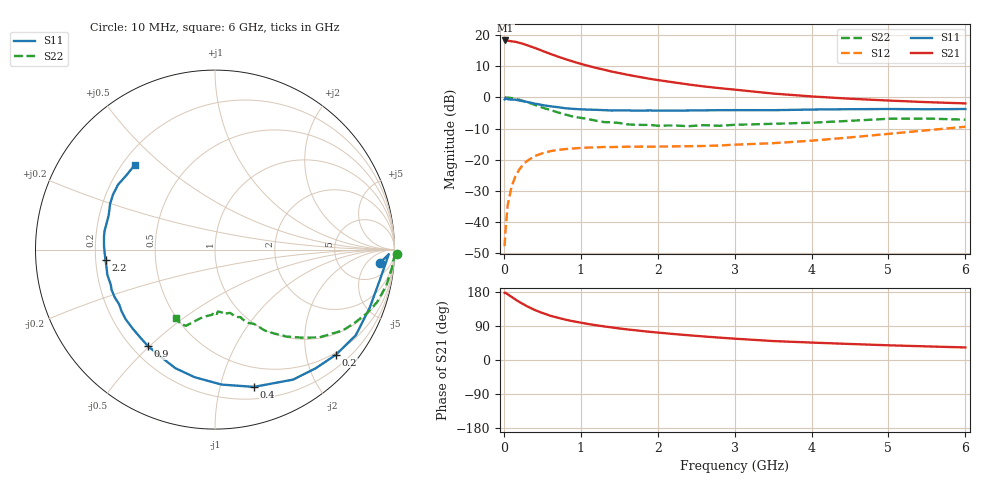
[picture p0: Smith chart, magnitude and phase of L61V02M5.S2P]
!  INFINEON TECHNOLOGIES Small Signal Semiconductors
! BFR380L3 , Si-NPN RF-Transistor in TSLP-3-1
!  Vce=1 V,  Ic=2.5 mA
! Common Emitter S-Parameters:  07. March 2005
#  GHz  S  MA  R  50
! f  S11  S21  S12  S22
! GHz  Mag  Ang  Mag  Ang  Mag  Ang  Mag  Ang
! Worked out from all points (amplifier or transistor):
!   36 points, 10 MHz to 6 GHz, reference 50 ohm
!   highest |S21| = 18.3 dB at 20 MHz (marker M1)
!   |S21| within 3 dB of that: start of sweep to 466.3 MHz
!   unconditionally stable (mu >= 1): 2.647 GHz to 4.82 GHz
!   at 250 MHz: K = 0.10, MSG = 19.4 dB, |S12| = -21.6 dB
!   at 1.4 GHz: K = 0.61, MSG = 12.1 dB, |S12| = -15.9 dB
!   at 6 GHz: K = 0.94, MSG = 3.7 dB, |S12| = -9.4 dB
!   S11 on the Smith chart (normalised r, x): 10 MHz: 13, -13; 200 MHz: 0.45, -2.61; 400 MHz: 0.31, -1.28; 900 MHz: 0.26, -0.49; 2.2 GHz: 0.24, -0.05; 6 GHz: 0.25, +0.41
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0.01  0.9239 -4.5  8.127 177.0  0.0041 84.9  1.013 -1.3
0.02  0.9687 -1.5  8.181 177.7  0.007 88.4  0.9989 -2.6
0.05  0.9335 -10.6  8.096 173.2  0.0187 84.8  0.9907 -6.1
0.1  0.9209 -20.6  7.929 166.6  0.0368 78.8  0.975 -11.9
0.15  0.918 -31.3  7.79 159.8  0.0539 73.1  0.9498 -17.9
0.2  0.8932 -40.9  7.512 153.3  0.0695 68.2  0.9178 -22.7
0.3  0.8451 -59.0  6.874 141.9  0.0951 58.7  0.8417 -32.4
0.4  0.7949 -74.2  6.225 132.2  0.1142 51.5  0.7594 -40.1
0.5  0.753 -87.2  5.583 124.2  0.1265 46.0  0.6878 -45.5
0.6  0.7199 -99.1  5.003 117.1  0.1369 41.2  0.6278 -50.5
0.7  0.6965 -108.5  4.518 111.6  0.1433 38.4  0.5755 -54.5
0.8  0.6693 -116.9  4.11 106.5  0.1481 35.7  0.531 -58.3
0.9  0.654 -125.0  3.748 102.2  0.1512 33.5  0.4904 -60.7
1.1  0.6355 -136.4  3.193 94.8  0.1565 31.0  0.4478 -65.6
1.3  0.6239 -146.6  2.784 88.7  0.16 29.8  0.4013 -69.4
1.6  0.6184 -158.8  2.314 80.8  0.1614 29.3  0.3697 -75.6
2.2  0.6128 -174.4  1.745 68.7  0.1635 32.4  0.3545 -82.9
2.8  0.6226 173.4  1.407 59.1  0.1688 38.7  0.3495 -91.6
3.5  0.6226 162.0  1.151 50.0  0.1841 45.7  0.3766 -98.5
4.5  0.6456 151.8  0.951 42.3  0.2278 55.8  0.4201 -106.5
5.5  0.6444 140.1  0.838 35.9  0.2965 59.7  0.4573 -114.7
6  0.6501 133.4  0.8 33.1  0.3379 59.5  0.4383 -119.7
